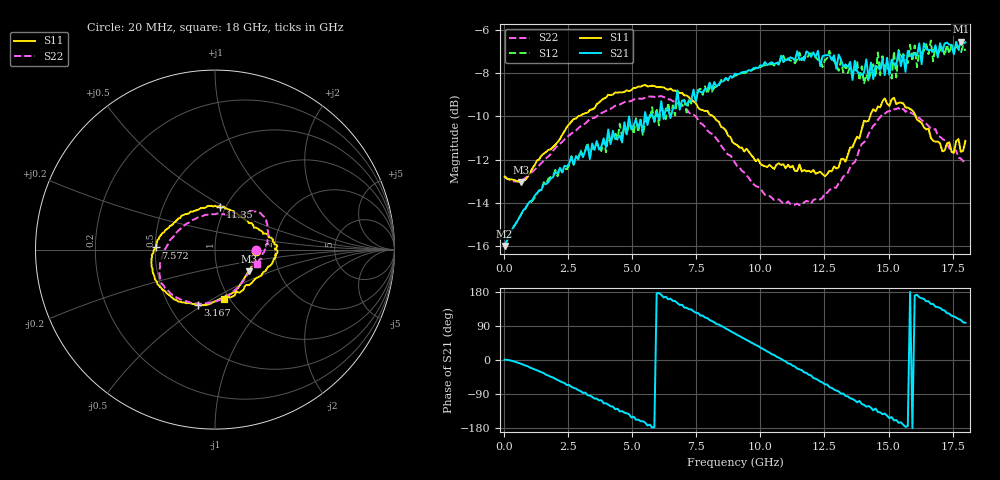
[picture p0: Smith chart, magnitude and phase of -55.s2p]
!Agilent Technologies,N5230A,US43500223,A.07.50.48
!Agilent N5230A: A.07.50.48
!Date: Thursday, January 14, 2016 15:05:28
!Correction: S11(Full 2 Port(1,2))
!S21(Full 2 Port(1,2))
!S12(Full 2 Port(1,2))
!S22(Full 2 Port(1,2))
!S2P File: Measurements: S11, S21, S12, S22:
# Hz S  dB  R 50
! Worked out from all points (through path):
!   201 points, 20 MHz to 18 GHz, reference 50 ohm
!   highest |S21| = -6.55 dB at 17.82 GHz (marker M1); lowest = -16.0 dB at 20 MHz (marker M2)
!   group delay of S21, straight-line fit = 98.7 ps
!   lowest |S11| = -13.0 dB at 649.3 MHz (marker M3), VSWR 1.57, Z = 70.4 - j17.9 ohm
!   |S11| at or under -10 dB: start of sweep to 2.888 GHz; 8.157 GHz to 14.28 GHz (6.124 GHz wide, 54.6 % of centre); 16.06 GHz to end of sweep
!   |S22| runs from -14.1 to -9.1 dB; largest |S21 - S12| = 0.066
!   S11 on the Smith chart (normalised r, x): 20 MHz: 1.59, -0.02; 3.167 GHz: 0.69, -0.47; 7.572 GHz: 0.50, +0.01; 11.35 GHz: 0.94, +0.47; 18 GHz: 0.95, -0.56
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2e7  -12.79 -1.7  -15.98 0.7  -15.99 0.5  -12.75 -1.1
6.493e8  -13.03 -32.8  -14.57 -9.7  -14.56 -9.9  -12.94 -30.8
1.9079e9  -11.41 -78.0  -12.80 -46.0  -12.75 -46.6  -11.60 -72.6
3.0766e9  -9.89 -106.0  -11.88 -87.0  -11.81 -87.0  -10.39 -98.8
3.1665e9  -9.86 -107.3  -11.61 -86.0  -11.58 -87.0  -10.33 -100.6
4.8746e9  -8.84 -139.1  -10.00 -142.9  -10.38 -143.8  -9.31 -129.7
6.0433e9  -8.65 -157.2  -10.14 176.4  -10.42 172.0  -9.08 -147.0
7.5716e9  -9.60 177.9  -8.79 123.8  -8.79 123.2  -10.15 -167.1
9.01e9  -11.28 146.9  -8.03 70.0  -8.13 67.9  -12.14 164.8
1.02686e10  -12.34 111.8  -7.64 22.3  -7.64 19.8  -13.65 130.7
1.13474e10  -12.51 83.6  -7.43 -17.3  -7.55 -21.3  -14.08 98.8
1.20666e10  -12.47 63.6  -7.05 -47.6  -7.12 -48.2  -13.86 77.8
1.26959e10  -12.51 46.2  -7.18 -71.7  -6.98 -72.6  -13.40 62.3
1.36848e10  -11.17 22.5  -7.44 -106.4  -7.89 -105.7  -12.11 51.5
1.45838e10  -9.55 6.7  -7.74 -137.3  -7.05 -137.9  -10.16 43.3
1.50333e10  -9.52 0.9  -8.09 -153.5  -7.90 -156.7  -9.75 37.9
1.55727e10  -9.40 -8.0  -7.15 -170.7  -7.12 -168.9  -9.65 29.5
1.58424e10  -9.66 -12.1  -7.21 179.5  -6.70 171.9  -9.81 25.6
1.63818e10  -10.50 -24.5  -6.63 161.2  -6.98 158.9  -10.22 15.9
1.7101e10  -11.62 -48.9  -7.01 132.4  -6.74 126.1  -11.04 1.3
1.78202e10  -11.64 -76.5  -6.55 105.8  -7.08 101.0  -11.95 -14.3
1.8e10  -11.13 -79.3  -6.59 98.2  -6.98 91.9  -12.10 -18.6
